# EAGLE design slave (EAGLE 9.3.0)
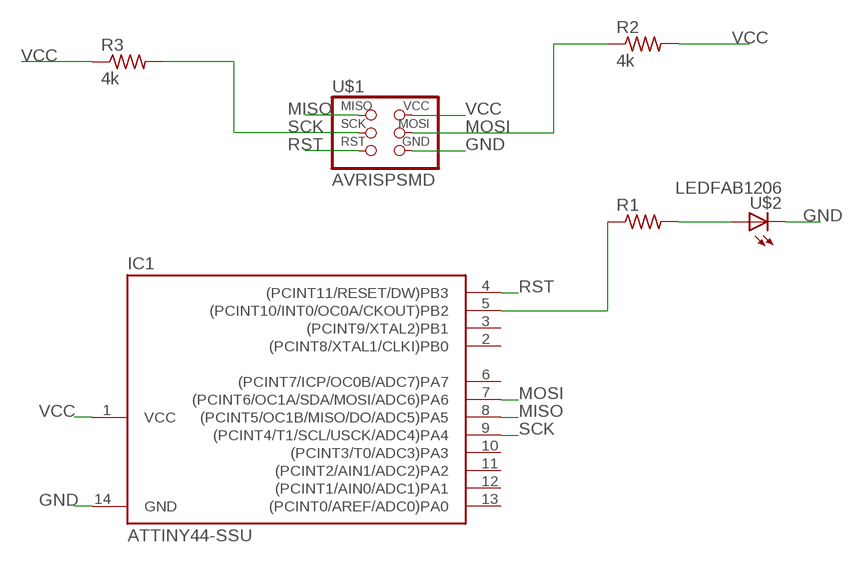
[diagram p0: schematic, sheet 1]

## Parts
IC1  ATTINY44-SSU  [SOIC14]
R1  RES-US1206FAB  [R1206FAB]
R2  4k  RES-US1206FAB  [R1206FAB]
R3  4k  RES-US1206FAB  [R1206FAB]
U$1  AVRISPSMD  [2X03SMD]
U$2  LEDFAB1206  [LED1206FAB]

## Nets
DELETE\DELETE: IC1.5((PCINT10/INT0/OC0A/CKOUT)PB2) R1.1
GND: IC1.14(GND) U$1.6(GND) U$2.2(C)
MISO: IC1.8((PCINT5/OC1B/MISO/DO/ADC5)PA5) U$1.1(MISO)
MOSI: IC1.7((PCINT6/OC1A/SDA/MOSI/ADC6)PA6) R2.1 U$1.4(MOSI)
N$1: R1.2 U$2.1(A)
RST: IC1.4((PCINT11/RESET/DW)PB3) U$1.5(RST)
SCK: IC1.9((PCINT4/T1/SCL/USCK/ADC4)PA4) R3.2 U$1.3(SCK)
VCC: IC1.1(VCC) R2.2 R3.1 U$1.2(VCC)
Unconnected: IC1.2((PCINT8/XTAL1/CLKI)PB0) IC1.3((PCINT9/XTAL2)PB1) IC1.6((PCINT7/ICP/OC0B/ADC7)PA7) IC1.10((PCINT3/T0/ADC3)PA3) IC1.11((PCINT2/AIN1/ADC2)PA2) IC1.12((PCINT1/AIN0/ADC1)PA1) IC1.13((PCINT0/AREF/ADC0)PA0)

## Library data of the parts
IC1 = fab:ATTINY44
R1-R3 = fab:RES-US: Resistor (US Symbol)
U$1 = fab:AVRISP
U$2 = fab:LED: LED

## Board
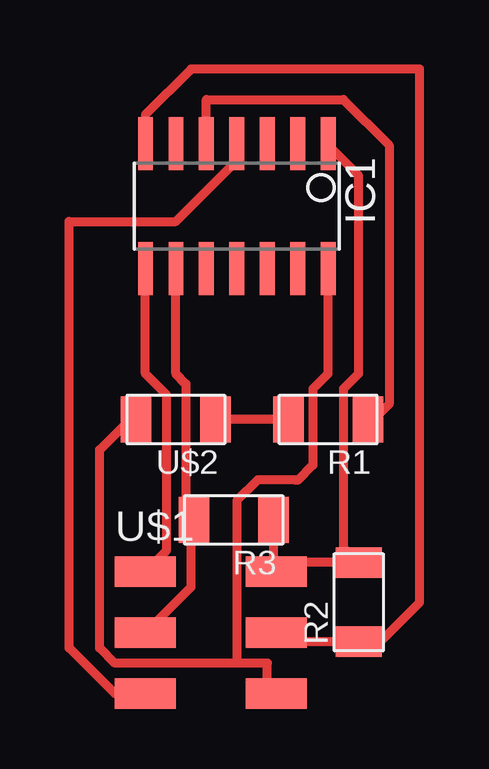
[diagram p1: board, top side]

No outline drawn. Coordinates in mm, seen from the top.
Copper layers (1*16): Top 0.035mm / dielectric 1.5mm / Bottom 0.035mm
Design rules "default *": minimum track width 15mil, minimum drill 0.35mm, track to track 15mil, track to pad 6mil, pad to pad 6mil, via to via 6mil, smd to smd 6mil, copper to edge 40mil, drill to drill 6mil, minimum pad ring 10mil, minimum via ring 8mil, stop-mask expansion 4mil, vias tented up to drill 0mil, thermal gap 10mil

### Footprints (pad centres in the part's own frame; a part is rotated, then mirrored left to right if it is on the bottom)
SOIC14 = smd 0.61 x 2.21: 1 -3.81,-2.603; 2 -2.54,-2.603; 3 -1.27,-2.603; 4 0,-2.603; 5 1.27,-2.603; 6 2.54,-2.603; 7 3.81,-2.603; 8 3.81,2.603; 9 2.54,2.603; 10 1.27,2.603; 11 0,2.603; 12 -1.27,2.603; 13 -2.54,2.603; 14 -3.81,2.603
R1206FAB = smd 1.27 x 1.905: 1 -1.651,0; 2 1.651,0
2X03SMD = smd 2.54 x 1.27: 1 -2.54,2.54; 2 2.92,2.54; 3 -2.54,0; 4 2.92,0; 5 -2.54,-2.54; 6 2.92,-2.54
LED1206FAB = smd 1.27 x 1.905: 1 -1.651,0; 2 1.651,0

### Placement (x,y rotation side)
IC1  64.77,49.53 180 top
R1  68.58,40.64 180 top
R2  69.85,33.02 90 top
R3  64.64,36.45 180 top
U$1  63.5,31.75 0 top
U$2  62.23,40.64 180 top

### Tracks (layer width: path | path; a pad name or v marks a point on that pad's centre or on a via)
DELETE\DELETE
  Top 0.381: IC1.5 63.5,53.98 69.22,53.98 71.12,52.07 71.12,41.27 70.48,40.64 R1.1
GND
  Top 0.381: 64.77,30.48 66.04,30.48 66.04,29.21 U$1.6 | 64.77,30.48 59.69,30.48 59.05,31.11 59.05,39.37 60.33,40.64 U$2.2 | IC1.14 68.58,42.55 67.94,41.91 67.94,38.73 67.31,38.1 67.22,38.1 67.2,38.12 65.64,38.12 64.77,37.25 64.77,30.48
MISO
  Top 0.381: IC1.8 60.96,42.55 61.85,41.66 61.85,35.18 U$1.1
MOSI
  Top 0.381: IC1.7 60.96,53.34 62.87,55.24 72.39,55.24 72.39,33.02 70.74,31.37 R2.1 67.06,31.37 66.67,31.75 U$1.4
N$1
  Top 0.381: R1.2 U$2.1
RST
  Top 0.381: IC1.4 64.77,51.44 62.23,48.9 57.78,48.9 57.78,31.11 59.69,29.21 U$1.5
SCK
  Top 0.381: IC1.9 62.23,42.55 62.65,42.13 62.65,37.17 62.99,36.83 R3.2 62.87,36.32 62.87,33.66 U$1.3
VCC
  Top 0.381: IC1.1 68.58,52.07 69.85,50.8 69.85,42.55 69.22,41.91 69.22,35.31 R2.2 67.06,34.67 66.67,34.29 U$1.2 66.29,34.42 R3.1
